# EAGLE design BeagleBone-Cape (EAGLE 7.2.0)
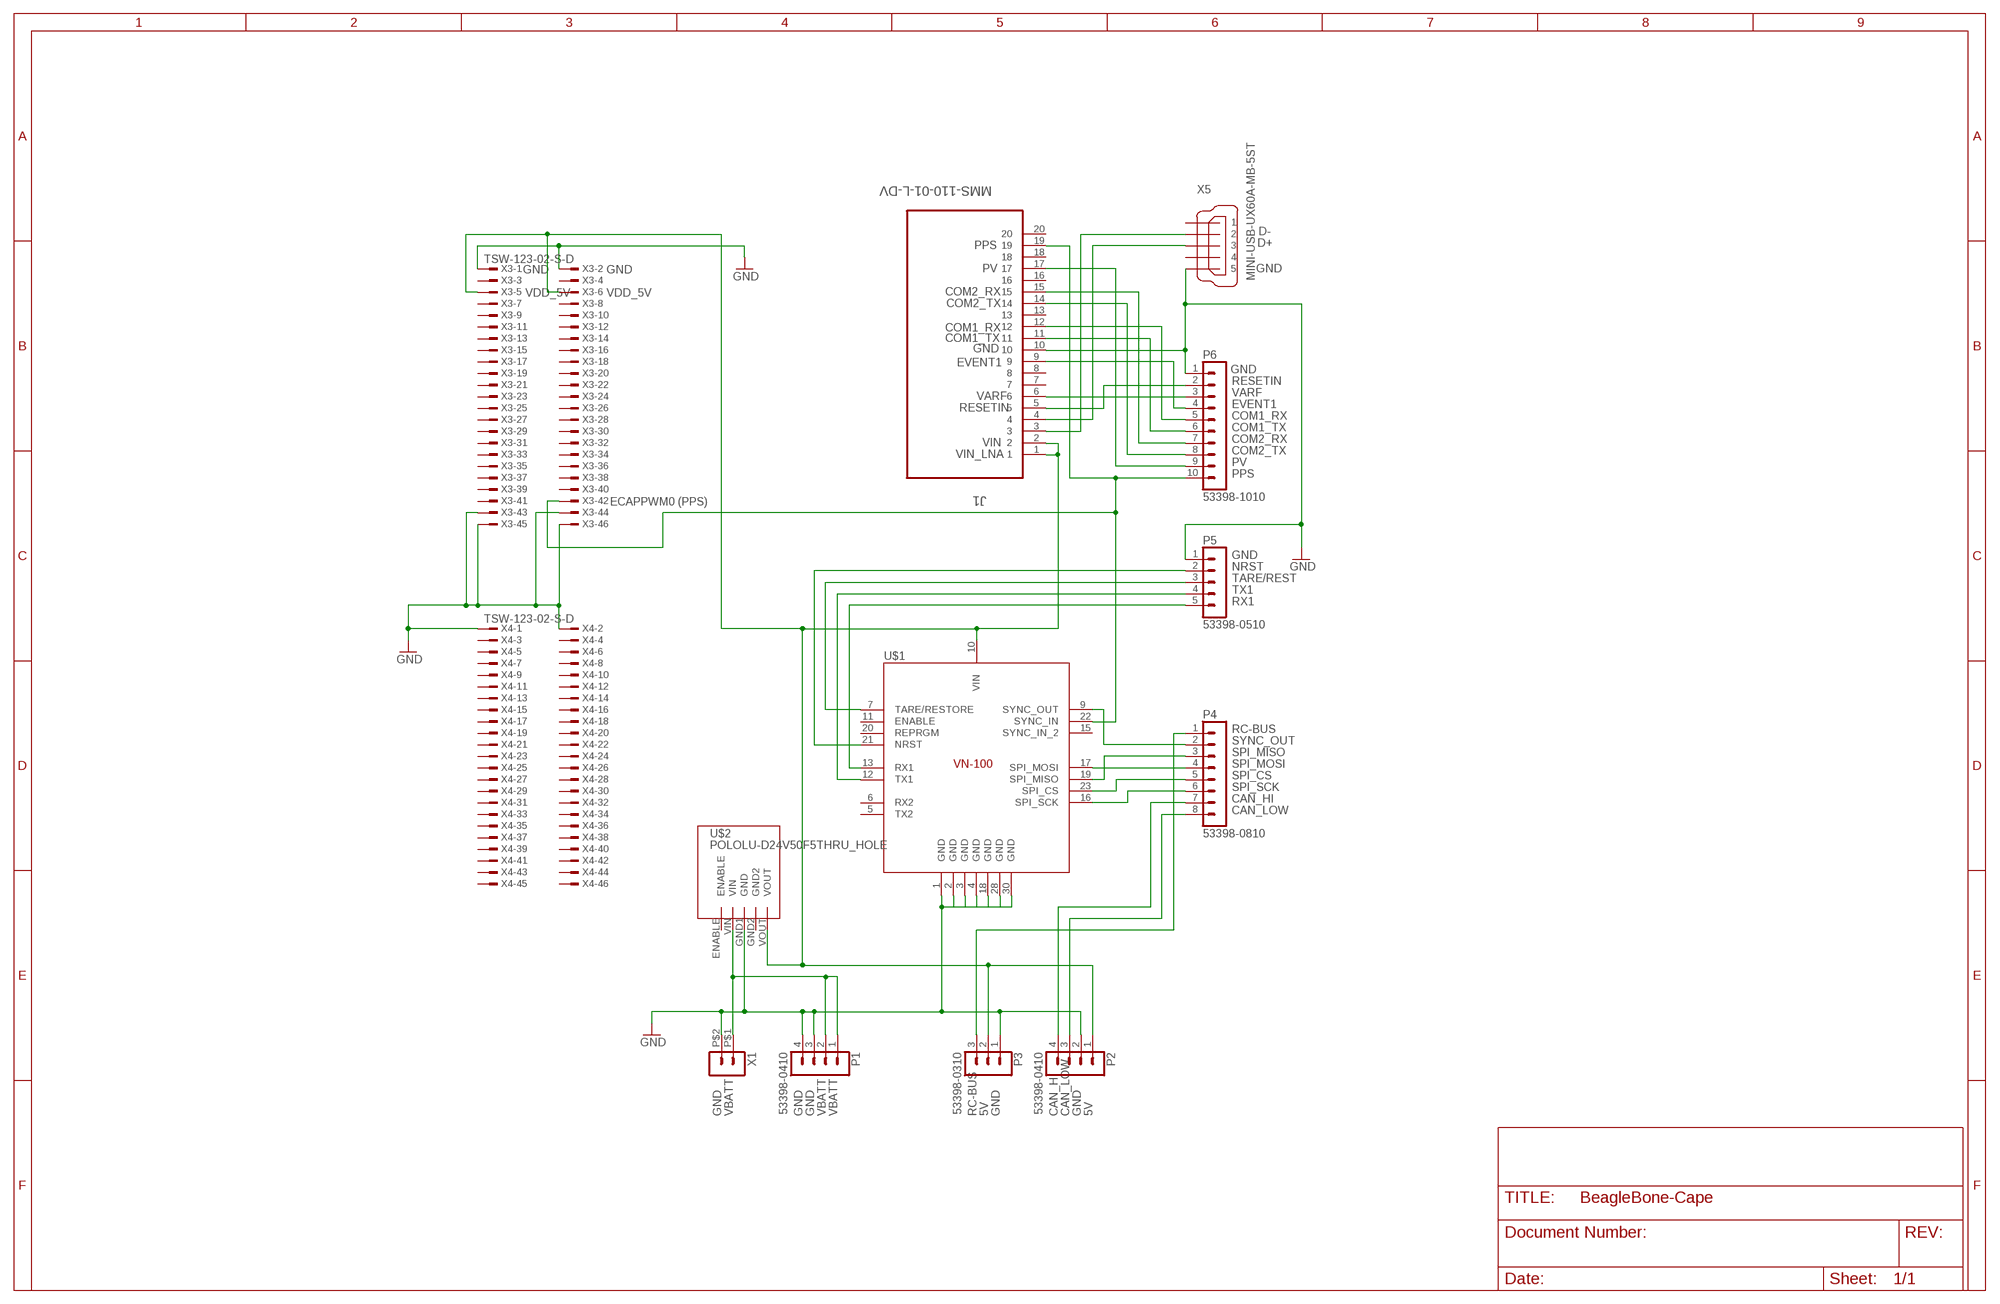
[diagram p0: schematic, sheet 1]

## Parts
J1  MMS-110-01-L-DV  [SAMTEC_MMS-110-01-L-DV]
P1  53398-0410  [53398-0410]
P2  53398-0410  [53398-0410]
P3  53398-0310  [53398-0310]
P4  53398-0810  [53398-0810]
P5  53398-0510  [53398-0510]
P6  53398-1010  [53398-1010]
U$1  VN100NORMAL  [7X8CASTLE]
U$2  POLOLU-D24V50F5THRU_HOLE  [POLOLU-D24V50F5]
X1  HEADER_POS2_  [43650-0203]
X3  TSW-123-02-S-D  [TSW-123-02-S-D]
X4  TSW-123-02-S-D  [TSW-123-02-S-D]
X5  MINI-USB-UX60A-MB-5ST  [UX60A-MB-5ST]

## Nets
GND: J1.10 P1.3 P1.4 P2.2 P3.1 P5.1 P6.1 U$1.1(GND) U$1.2(GND) U$1.3(GND) U$1.4(GND) U$1.18(GND) U$1.28(GND) U$1.30(GND) U$2.GND1(GND) X1.P$2 X3.1 X3.2 X3.43 X3.44 X3.45 X3.46 X4.1 X4.2 X5.5
N$1: P1.1 P1.2 U$2.VIN X1.P$1
N$2: J1.19 P6.10 U$1.22(SYNC_IN) X3.42
N$3: J1.1 J1.2 P2.1 P3.2 U$1.10(VIN) U$2.VOUT X3.5 X3.6
N$4: P5.5 U$1.13(RX1)
N$5: P3.3 P4.1
N$6: P2.3 P4.8
N$7: P2.4 P4.7
N$8: P5.4 U$1.12(TX1)
N$9: P4.2 U$1.9(SYNC_OUT)
N$10: P4.3 U$1.19(SPI_MISO)
N$11: P5.3 U$1.7(TARE/RESTORE)
N$12: P5.2 U$1.21(NRST)
N$13: J1.3 X5.2
N$14: P4.4 U$1.17(SPI_MOSI)
N$15: P4.5 U$1.23(SPI_CS)
N$16: P4.6 U$1.16(SPI_SCK)
N$20: J1.4 X5.3
N$21: J1.5 P6.2
N$23: J1.6 P6.3
N$24: J1.9 P6.4
N$25: J1.12 P6.5
N$26: J1.11 P6.6
N$27: J1.15 P6.7
N$28: J1.14 P6.8
N$29: J1.17 P6.9
Unconnected: J1.7 J1.8 J1.13 J1.16 J1.18 J1.20 U$1.5(TX2) U$1.6(RX2) U$1.11(ENABLE) U$1.15(SYNC_IN_2) U$1.20(REPRGM) U$2.ENABLE U$2.GND2 X3.3 X3.4 X3.7 X3.8 X3.9 X3.10 X3.11 X3.12 X3.13 X3.14 X3.15 X3.16 X3.17 X3.18 X3.19 X3.20 X3.21 X3.22 X3.23 X3.24 X3.25 X3.26 X3.27 X3.28 X3.29 X3.30 X3.31 X3.32 X3.33 X3.34 X3.35 X3.36 X3.37 X3.38 X3.39 X3.40 X3.41 X4.3 X4.4 X4.5 X4.6 X4.7 X4.8 X4.9 X4.10 X4.11 X4.12 X4.13 X4.14 X4.15 X4.16 X4.17 X4.18 X4.19 X4.20 X4.21 X4.22 X4.23 X4.24 X4.25 X4.26 X4.27 X4.28 X4.29 X4.30 X4.31 X4.32 X4.33 X4.34 X4.35 X4.36 X4.37 X4.38 X4.39 X4.40 X4.41 X4.42 X4.43 X4.44 X4.45 X4.46 X5.1 X5.4

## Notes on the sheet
- D-
- PPS | D+
- GND | GND | PV | GND
- VDD_5V | VDD_5V | COM2_RX
- COM2_TX
- COM1_RX
- COM1_TX
- GND
- EVENT1
- GND
- RESETIN
- VARF
- VARF
- EVENT1
- RESETIN
- COM1_RX
- COM1_TX
- COM2_RX
- VIN
- COM2_TX
- VIN_LNA
- PV
- PPS
- ECAPPWM0 (PPS)
- GND
- NRST
- TARE/REST
- TX1
- RX1
- RC-BUS
- SYNC_OUT
- SPI_MISO
- SPI_MOSI
- SPI_CS
- SPI_SCK
- CAN_HI
- CAN_LOW
- GND | VBATT | GND | GND | VBATT | VBATT | RC-BUS | 5V | GND | CAN_HI | CAN_LOW | GND | 5V

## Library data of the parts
J1 = SAMTEC-FLE-Mxx-Sxx_By_element14_Batch_1:MMS-110-01-L-DV: CONN RECEPTACLE, 2MM, VERT, 20WAY; MPN: MMS-110-01-L-DV; OC_FARNELL: 1667856; OC_NEWARK: 11P5392; PACKAGE: RECEPTACLE, 2MM, VERT, 20WAY; SUPPLIER: Samtec
P1 P2 = con-molex-picoblade:53398-0410: HEADER
P3 = con-molex-picoblade:53398-0310: HEADER
P4 = con-molex-picoblade:53398-0810: HEADER
P5 = con-molex-picoblade:53398-0510: HEADER
P6 = con-molex-picoblade:53398-1010: HEADER
U$1 = vectornav:VN100: VectorNav VN-100(T) Inertial Measurement Unit (IMU) and Attitude Heading Reference System (AHRS).
U$2 = pololu-D24V50F5:POLOLU-D24V50F5
X1 = con-molex-micro-fit-3_0:HEADER_POS2_?: Molex - Micro-Fit 3.0 Series connector, 3.00mm (0.118") pitch header, 2 positions.
X3 X4 = con-samtec:TSW-123-02-S-D: THROUGH-HOLE .025" SQ POST HEADER Source: Samtec TSW.pdf; OC_FARNELL: unknown; OC_NEWARK: unknown
X5 = con-hirose:MINI-USB-: MINI USB Connector Source: http://www.hirose.co.jp/cataloge_hp/e24000019.pdf; OC_FARNELL: unknown; OC_NEWARK: unknown

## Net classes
0 default: width 0.254 mm, drill 0.584 mm, clearance 0.254 mm

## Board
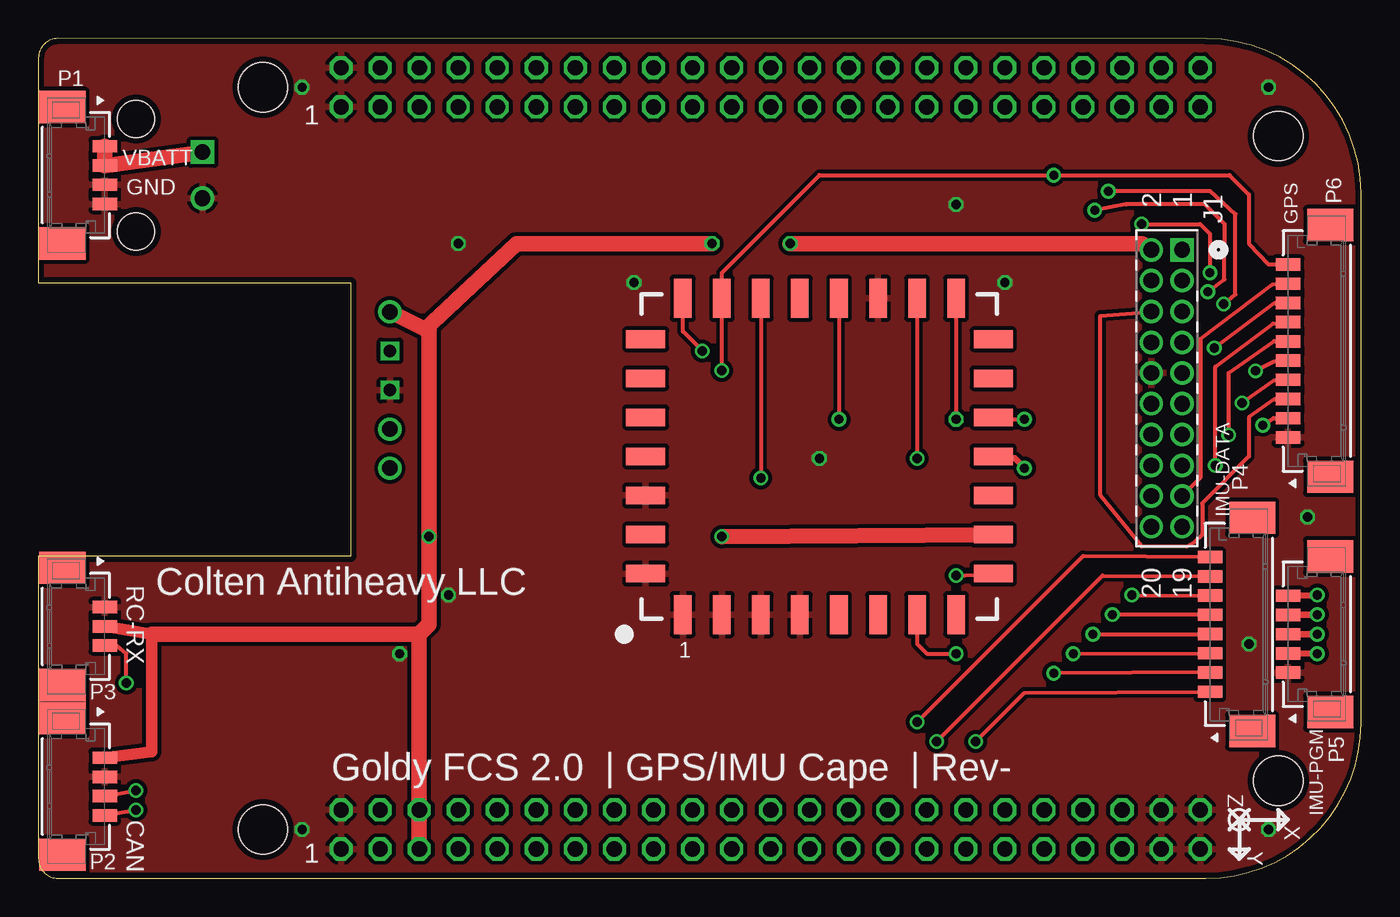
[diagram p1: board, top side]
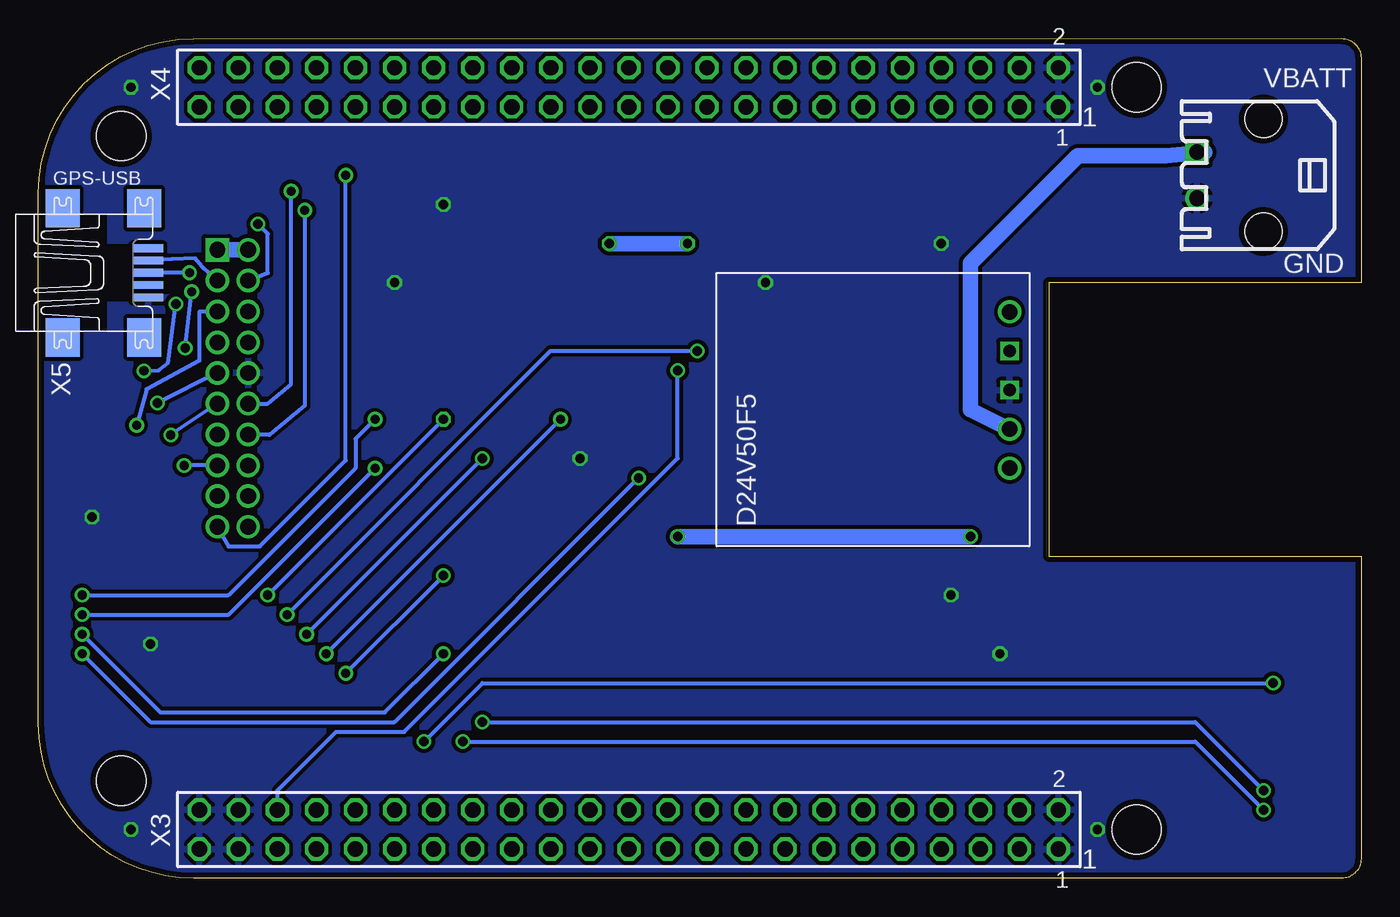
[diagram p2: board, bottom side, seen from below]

Size 86.03 x 54.61 mm. Coordinates in mm from the lower left corner, seen from the top.
Outline: 0,20.95 0,1.27 arc90 1.27,0 75.95,0 arc90 86.03,10.08 86.03,44.53 arc90 75.96,54.6 1.27,54.61 arc90 0,53.34 0,38.73 20.32,38.73 20.32,20.95 0,20.95
Copper layers (1*16): Top 0.0356mm / dielectric 1.5011mm / Bottom 0.0356mm
Design rules "oshpark-2layer *": minimum track width 6mil, minimum drill 13mil, track to track 6mil, track to pad 6mil, pad to pad 6mil, via to via 6mil, smd to smd 6mil, copper to edge 15mil, drill to drill 6mil, minimum pad ring 7mil, minimum via ring 7mil, stop-mask expansion 4mil, vias tented up to drill 25mil, thermal gap 10mil
Holes 3.2 mm at 14.61,3.17 14.61,51.44 80.64,6.35 80.64,48.26

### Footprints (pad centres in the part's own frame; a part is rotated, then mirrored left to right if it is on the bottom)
SAMTEC_MMS-110-01-L-DV = drill 1.016 square: 1 18.009,-2.007 | drill 1.016: 2 18.009,0; 3 16.002,-2.007; 4 16.002,0; 5 13.995,-2.007; 6 13.995,0; 7 11.989,-2.007; 8 11.989,0; 9 10.008,-2.007; 10 10.008,0; 11 8.001,-2.007; 12 8.001,0; 13 5.994,-2.007; 14 5.994,0; 15 3.988,-2.007; 16 3.988,0; 17 2.007,-2.007; 18 2.007,0; 19 0,-2.007; 20 0,0
53398-0410 = smd 0.8 x 1.6: 1 1.875,0; 2 0.625,0; 3 -0.625,0; 4 -1.875,0 | smd 2.1 x 3: M1 4.435,2.75; M2 -4.435,2.75
53398-0310 = smd 0.8 x 1.6: 1 1.25,0; 2 0,0; 3 -1.25,0 | smd 2.1 x 3: M1 3.81,2.75; M2 -3.81,2.75
53398-0810 = smd 0.8 x 1.6: 1 4.375,0; 2 3.125,0; 3 1.875,0; 4 0.625,0; 5 -0.625,0; 6 -1.875,0; 7 -3.125,0; 8 -4.375,0 | smd 2.1 x 3: M1 6.935,2.75; M2 -6.935,2.75
53398-0510 = smd 0.8 x 1.6: 1 2.5,0; 2 1.25,0; 3 0,0; 4 -1.25,0; 5 -2.5,0 | smd 2.1 x 3: M1 5.06,2.75; M2 -5.06,2.75
53398-1010 = smd 0.8 x 1.6: 1 5.625,0; 2 4.375,0; 3 3.125,0; 4 1.875,0; 5 0.625,0; 6 -0.625,0; 7 -1.875,0; 8 -3.125,0; 9 -4.375,0; 10 -5.625,0 | smd 2.1 x 3: M1 8.185,2.75; M2 -8.185,2.75
7X8CASTLE = smd 2.54 x 1.143: 1 10.16,-8.89; 2 10.16,-6.35; 3 10.16,-3.81; 4 10.16,-1.27; 5 10.16,1.27; 6 10.16,3.81; 7 10.16,6.35; 8 10.16,8.89; 16 -10.414,8.89; 17 -10.414,6.35; 18 -10.414,3.81; 19 -10.414,1.27; 20 -10.414,-1.27; 21 -10.414,-3.81; 22 -10.414,-6.35; 23 -10.414,-8.89 | smd 1.143 x 2.54: 9 7.493,11.303; 10 4.953,11.303; 11 2.413,11.303; 12 -0.127,11.303; 13 -2.667,11.303; 14 -5.207,11.303; 15 -7.747,11.303; 24 -7.747,-11.303; 25 -5.207,-11.303; 26 -2.667,-11.303; 27 -0.127,-11.303; 28 2.413,-11.303; 29 4.953,-11.303; 30 7.493,-11.303
POLOLU-D24V50F5 = drill 1: ENABLE 0,0; VIN 2.54,0; VOUT 10.16,0 | drill 0.8 square: GND1 5.08,0; GND2 7.62,0
43650-0203 = drill 1.02 square: P$1 1.5,4.32 | drill 1.02: P$2 -1.5,4.32 | hole 2.413: 3.658,0; -3.658,0
TSW-123-02-S-D = drill 1 pad 1.5 octagon: 1 27.94,-1.27; 2 27.94,1.27; 3 25.4,-1.27; 4 25.4,1.27; 5 22.86,-1.27; 6 22.86,1.27; 7 20.32,-1.27; 8 20.32,1.27; 9 17.78,-1.27; 10 17.78,1.27; 11 15.24,-1.27; 12 15.24,1.27; 13 12.7,-1.27; 14 12.7,1.27; 15 10.16,-1.27; 16 10.16,1.27; 17 7.62,-1.27; 18 7.62,1.27; 19 5.08,-1.27; 20 5.08,1.27; 21 2.54,-1.27; 22 2.54,1.27; 23 0,-1.27; 24 0,1.27; 25 -2.54,-1.27; 26 -2.54,1.27; 27 -5.08,-1.27; 28 -5.08,1.27; 29 -7.62,-1.27; 30 -7.62,1.27; 31 -10.16,-1.27; 32 -10.16,1.27; 33 -12.7,-1.27; 34 -12.7,1.27; 35 -15.24,-1.27; 36 -15.24,1.27; 37 -17.78,-1.27; 38 -17.78,1.27; 39 -20.32,-1.27; 40 -20.32,1.27; 41 -22.86,-1.27; 42 -22.86,1.27; 43 -25.4,-1.27; 44 -25.4,1.27; 45 -27.94,-1.27; 46 -27.94,1.27
UX60A-MB-5ST = smd 2 x 0.5: 1 2.25,1.6; 2 2.25,0.8; 3 2.25,0; 4 2.25,-0.8; 5 2.25,-1.6 | smd 2.2 x 2.5: M1 -3.3,-4.2; M2 -3.3,4.2; M3 2,4.2; M4 2,-4.2

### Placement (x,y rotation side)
J1  72.39,22.86 90 top
P1  4.32,45.72 90 top
P2  4.32,5.97 90 top
P3  4.32,16.38 90 top
P4  76.2,16.51 270 top
P5  81.28,15.88 270 top
P6  81.28,34.29 270 top
U$1  50.8,27.3 270 top
U$2  22.86,26.67 90 bottom
X1  6.35,45.72 90 bottom
X3  47.62,3.17 0 bottom
X4  47.62,51.44 0 bottom
X5  81.15,39.37 0 bottom

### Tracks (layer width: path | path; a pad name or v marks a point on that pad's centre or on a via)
GND  (via drill 0.6)
  other vias: 82.55,23.5 80.01,3.17 80.01,51.44 17.14,51.44 17.14,3.17 50.8,27.3 26.67,18.41 27.3,41.27 38.73,38.73 78.74,15.24 59.69,43.81 23.5,14.61 62.87,38.73
  pour Top: -1.27,55.88 -1.27,-1.27 87.63,-1.27 87.63,55.88
  pour Bottom: -1.27,55.88 87.63,55.88 87.63,-1.27 -1.27,-1.27
N$1
  Top 1.016: P1.1 P1.2 X1.P$1
  Bottom 0.61: 10.16,47.22 X1.P$1
  Bottom 1.016: U$2.VIN 25.4,30.48 25.4,40.01 18.41,46.99 12.7,46.99 10.16,47.22
N$2  (via drill 0.6)
  Top 0.254: P6.10 80.01,39.91 78.74,41.27 78.74,44.45 77.47,45.72 v66.04,45.72 50.8,45.72 44.45,39.37 U$1.22 v44.45,33.02
  Bottom 0.254: J1.19 73.66,21.59 71.63,21.59 66.04,27.18 v66.04,45.72 | X3.42 70.48,5.71 66.67,9.53 62.23,9.53 44.45,27.3 v44.45,33.02
N$3  (via drill 0.6)
  Top 0.762: P2.1 7.37,8.22 7.37,15.88 P3.2
  Top 1.016: 7.37,15.88 24.77,15.88 | 24.77,15.88 25.4,16.51 v25.4,22.23 25.4,35.56 25.15,35.69 | 25.15,35.69 U$2.VOUT | U$1.10 v44.45,22.23 | J1.2 71.75,41.27 v48.9,41.27 | v43.81,41.27 31.11,41.27 25.15,35.69 | X3.5 X3.6 24.77,15.88
  Bottom 1.016: J1.1 J1.2 | v25.4,22.23 v44.45,22.23 | v48.9,41.27 v43.81,41.27
N$4  (via drill 0.6)
  Top 0.254: 62.87,29.84 v64.14,29.84
  Top 0.406: P5.5 v83.19,18.41 | U$1.13 62.87,29.84
  Bottom 0.254: v83.19,18.41 73.66,18.41 65.41,26.67 65.41,28.57 v64.14,29.84
N$5  (via drill 0.6, 0.61)
  Top 0.254: v5.71,12.7 5.71,14.61 5.08,15.11 P3.3 | v60.96,8.89 64.14,12.06 P4.1
  Bottom 0.254: v5.71,12.7 57.15,12.7 v60.96,8.89
N$6  (via drill 0.6)
  Top 0.254: P2.3 v6.35,5.71 | v57.15,10.16 67.94,20.95 P4.8
  Bottom 0.254: v57.15,10.16 10.79,10.16 v6.35,5.71
N$7  (via drill 0.6)
  Top 0.254: P2.4 v6.35,4.45 | v58.42,8.89 69.22,19.68 P4.7
  Bottom 0.254: v58.42,8.89 10.79,8.89 v6.35,4.45
N$8  (via drill 0.6)
  Top 0.406: P5.4 v83.19,17.14 | U$1.12 63.5,27.3 v64.14,26.67
  Bottom 0.254: v83.19,17.14 73.66,17.14 v64.14,26.67
N$9  (via drill 0.6)
  Top 0.254: P4.2 v66.04,13.34 | v59.69,19.68 U$1.9
  Bottom 0.254: v66.04,13.34 v59.69,19.68
N$10  (via drill 0.6)
  Top 0.254: U$1.19 v52.07,29.84 | v67.31,14.61 P4.3
  Bottom 0.254: v52.07,29.84 v67.31,14.61
N$11  (via drill 0.6)
  Top 0.254: U$1.7 57.15,15.24 57.78,14.61 v59.69,14.61
  Top 0.406: P5.3 v83.19,15.88
  Bottom 0.254: v83.19,15.88 78.11,10.79 63.5,10.79 v59.69,14.61
N$12  (via drill 0.6)
  Top 0.254: U$1.21 v46.99,26.04
  Top 0.406: P5.2 v83.19,14.61
  Bottom 0.254: v83.19,14.61 78.74,10.16 62.87,10.16 v46.99,26.04
N$13
  Bottom 0.254: J1.3 75.39,39.78 75.84,40.31 77.34,40.26 X5.2
N$14  (via drill 0.6)
  Top 0.254: U$1.17 v57.15,27.3 | v68.58,15.88 P4.4
  Bottom 0.254: v57.15,27.3 v68.58,15.88
N$15  (via drill 0.6)
  Top 0.254: P4.5 v69.85,17.14 | v43.18,34.29 41.91,35.56 U$1.23
  Bottom 0.254: v69.85,17.14 52.7,34.29 v43.18,34.29
N$16  (via drill 0.6)
  Top 0.254: U$1.16 v59.69,29.84 | v71.12,18.41 P4.6
  Bottom 0.254: v59.69,29.84 v71.12,18.41
N$20  (via drill 0.6)
  Top 0.254: v71.75,42.55 75.56,42.55 76.2,41.91 v76.2,39.37
  Bottom 0.254: J1.4 71.12,39.37 71.12,41.91 v71.75,42.55 | v76.2,39.37 X5.3
N$21  (via drill 0.6)
  Top 0.254: v79.64,29.46 80.34,29.92 P6.2
  Bottom 0.254: J1.5 75.56,36.83 75.56,33.66 78.99,31.8 v79.64,29.46
N$23
  Top 0.254: P6.3 80.39,31.14 78.74,29.97 78.74,27.43 75.69,24.38 75.69,22.35 75.18,21.84 74.68,21.57 71.75,21.59 69.09,24.89 69.09,36.58 J1.6
N$24  (via drill 0.6)
  Top 0.254: v78.28,30.91 80.37,32.38 P6.4
  Bottom 0.254: J1.9 v78.28,30.91
N$25  (via drill 0.6)
  Top 0.254: v69.6,44.68 70.1,44.7 76.2,44.7 77.85,43.18 77.85,37.97 v77.09,37.34 | P6.5 80.37,33.6 v79.17,32.99
  Bottom 0.254: J1.12 71.12,30.86 69.6,32.13 v69.6,44.68 | v79.17,32.99 78.23,33.02 77.6,33.53 v77.09,37.34
N$26  (via drill 0.6)
  Top 0.254: v77.42,28.83 77.42,32.87 80.37,34.92 P6.6
  Bottom 0.254: J1.11 v77.42,28.83
N$27  (via drill 0.6)
  Top 0.254: v76.56,26.85 76.56,33.27 80.29,36.07 P6.7
  Bottom 0.254: J1.15 v76.56,26.85
N$28  (via drill 0.6)
  Top 0.254: P6.8 80.69,37.41 80.39,37.39 v76.48,34.48 | v76.06,38.14 77.14,38.94 77.15,42.55 75.88,43.81 70.74,43.81 v68.71,43.43
  Bottom 0.254: v76.48,34.48 v76.06,38.14 | v68.71,43.43 68.71,30.73 70.99,28.83 J1.14
N$29
  Top 0.254: P6.9 80.26,38.61 75.56,35.05 75.56,26.04 J1.17

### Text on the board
_tsilk: 1 | VBATT | GND | GPS | IMU-DATA | RC-RX | Colten Antiheavy LLC | 1 | Goldy FCS 2.0 | GPS/IMU Cape | Rev- | Z | CAN | IMU-PGM | X | Y | 1
_bsilk: VBATT | 1 | GPS-USB | GND | 1

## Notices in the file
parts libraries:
con-molex-picoblade: Copyright (C) 2010, Bob Starr
